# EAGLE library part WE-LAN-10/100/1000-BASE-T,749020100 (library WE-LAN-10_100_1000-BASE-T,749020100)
LAN-Transformer WE-LAN 10/10/1000 Base Tx - Compliant with IEEE 802.3 standards - SMD -- Ethernet -- Power over Ethernet -- 1 Gigabit Ethernet -- Compliant with most IC's for ethernet applications like Intel, AMD, Globespan and Realtek -- Hub, Router, Switch
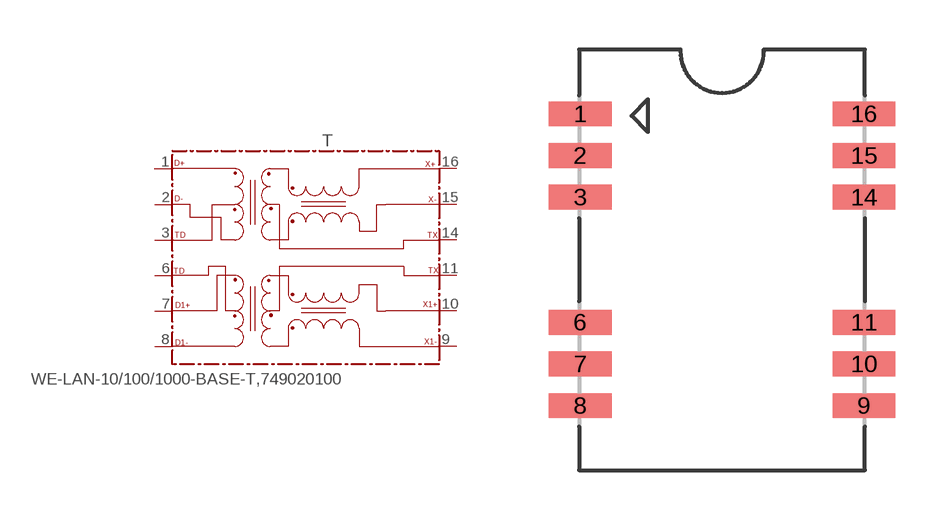
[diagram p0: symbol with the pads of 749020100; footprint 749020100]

Designator prefix T

## WE-LAN-10/100/1000-BASE-T,749020100 (MPN: 749020100; OC_FARNELL: 1636359; OC_NEWARK: 08P2951; PACKAGE: 10/100/1000/Base-T; SUPPLIER: Wuerth Elektronik)  [749020100]
1  D+
2  D-
3  TD1
6  TD2
7  D1+
8  D1-
9  X1-
10  X1+
11  TX1
14  TX
15  X-
16  X+

## Footprint 749020100 (pad centres in mm)
MAX Height = 2.16mm
smd 1.91 x 0.76: 1 -4.32,4.445; 2 -4.32,3.175; 3 -4.32,1.905; 6 -4.32,-1.905; 7 -4.32,-3.175; 8 -4.32,-4.445; 9 4.32,-4.445; 10 4.32,-3.175; 11 4.32,-1.905; 14 4.32,1.905; 15 4.32,3.175; 16 4.32,4.445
